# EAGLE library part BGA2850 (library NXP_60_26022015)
Silicon Monolithic Microwave Integrated Circuit (MMIC) wideband amplifier with internal matching circuit in a 6-pin SOT363 plastic SMD package. AAL Eindhoven MV+ MK
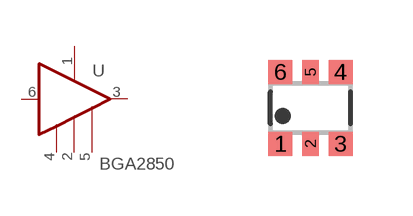
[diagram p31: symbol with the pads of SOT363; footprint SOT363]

Designator prefix U

## BGA2850 (12NC: 9352 900 54115)  [SOT363]
1  VCC  pwr
2  GND2  pwr
3  OUT  out
4  GND1  pwr
5  GND2  pwr
6  -IN  in

## Footprint SOT363 (pad centres in mm)
SOT363 Plastic surface-mounted package; 6 leads JEDEC: -- IEC: -- JEITA: SC-88
smd 0.6 x 0.6: 1 -0.75,-0.9; 3 0.75,-0.9; 4 0.75,0.9; 6 -0.75,0.9
smd 0.4 x 0.6: 2 0,-0.9; 5 0,0.9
